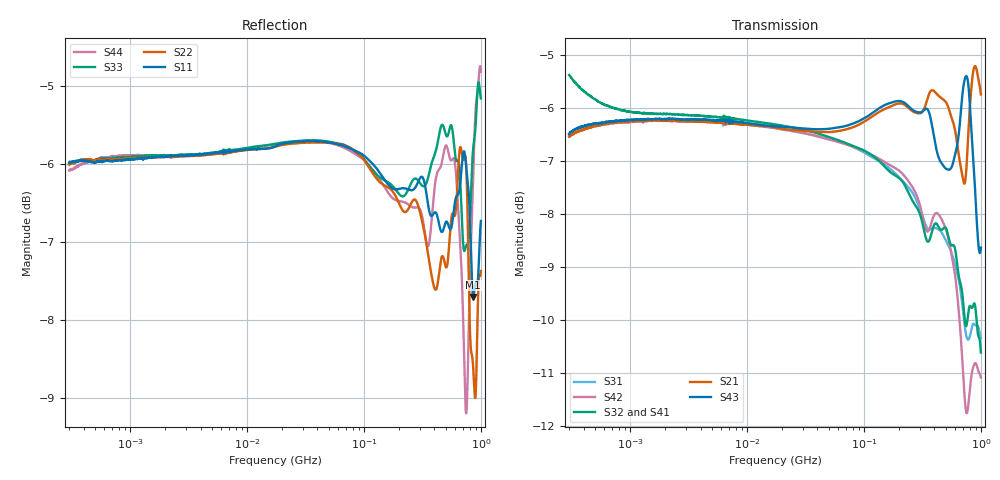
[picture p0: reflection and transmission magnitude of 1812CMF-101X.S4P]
!s-Parameter Generated by FASTRON Sdn. Bhd.
!FASTRON P/N : 1812CMF-101X
!Keysight Technologies: E5071C_MY46733604_B.14.02
!Date: Mon Mar 09 12:42:55 2026
!Version  :Rev00  Mon Mar 09 12:42:55 2026
!Data & Calibration Information:
!Freq	S11:SOLT4(ON)	S12:SOLT4(ON)	S13:SOLT4(ON)	S14:SOLT4(ON)
!	S21:SOLT4(ON)	S22:SOLT4(ON)	S23:SOLT4(ON)	S24:SOLT4(ON)
!	S31:SOLT4(ON)	S32:SOLT4(ON)	S33:SOLT4(ON)	S34:SOLT4(ON)
!	S41:SOLT4(ON)	S42:SOLT4(ON)	S43:SOLT4(ON)	S44:SOLT4(ON)
!PortZ  Port1:50+j0  Port2:50+j0  Port3:50+j0  Port4:50+j0
!When reading reference impedance value at option line is always used.
! Remarks : This data is being provided solely for informational purposes.
# Hz S dB R 50
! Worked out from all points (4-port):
!   1601 points, 300 kHz to 1 GHz, reference 50 ohm
!   strongest paths, dB at 300 kHz, 2.303 MHz, 17.55 MHz, 132.8 MHz, 1 GHz:
!     S43: -6.5, -6.2, -6.3, -6.0, -8.6
!     S21: -6.5, -6.2, -6.4, -6.1, -5.7
!     S32: -5.4, -6.1, -6.3, -7.0, -10.6
!     S41: -5.3, -6.1, -6.3, -7.0, -11.2
!     S42: -6.5, -6.2, -6.4, -6.9, -11.1
!     S31: -6.5, -6.2, -6.4, -7.0, -10.3
!   lowest |S11| = -7.7 dB at 861.1 MHz (marker M1), VSWR 2.40, Z = 120 - j3.58 ohm
!   |S11| at or under -10 dB: nowhere
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300000  -5.98 12.5  -6.57 14.6  -6.54 -165.6  -5.43 -13.5
        -6.54 14.3  -6.01 12.9  -5.37 -13.5  -6.60 -165.5
        -6.52 -165.8  -5.38 -13.5  -6.00 12.8  -6.59 14.6
        -5.33 -13.8  -6.51 -165.8  -6.49 14.3  -6.08 13.7
6.067004e7  -5.75 -4.4  -6.42 0.3  -6.61 152.8  -6.60 -27.2
            -6.43 0.3  -5.74 -6.1  -6.59 -28.0  -6.65 151.7
            -6.63 152.7  -6.61 -28.0  -5.73 -4.9  -6.40 0.4
            -6.59 -27.3  -6.64 151.6  -6.36 0.4  -5.76 -5.3
2.150325e8  -6.31 -10.5  -5.91 -3.1  -7.36 89.4  -7.47 -90.9
            -5.92 -3.0  -6.60 -15.0  -7.38 -92.7  -7.26 86.4
            -7.38 89.5  -7.40 -92.6  -6.41 -10.7  -5.90 -3.5
            -7.47 -90.7  -7.25 86.4  -5.88 -3.7  -6.48 -12.0
4.296107e8  -6.70 -12.5  -5.74 -8.7  -8.26 7.1  -8.25 -174.7
            -5.76 -8.6  -7.51 -17.7  -8.22 -176.4  -8.00 5.7
            -8.28 7.1  -8.22 -176.4  -5.70 -12.2  -6.89 -9.4
            -8.25 -174.6  -7.99 5.8  -6.90 -9.5  -6.09 -11.9
6.319272e8  -6.40 -4.3  -6.72 -15.1  -9.11 -74.8  -8.78 101.8
            -6.73 -15.0  -6.23 -13.6  -9.00 102.7  -9.58 -77.0
            -9.14 -74.8  -9.01 102.6  -5.96 -16.4  -6.62 -2.1
            -8.78 101.9  -9.58 -76.9  -6.66 -2.2  -6.44 -20.8
8.611227e8  -7.71 -1.7  -5.28 -10.5  -10.05 -158.5  -10.40 23.6
            -5.30 -10.4  -8.63 -9.4  -9.72 26.1  -10.90 -155.2
            -10.07 -158.5  -9.72 25.9  -5.78 2.5  -6.97 -19.0
            -10.43 23.8  -10.88 -155.1  -6.96 -19.0  -6.14 4.1
1e9  -6.73 11.3  -5.73 -21.7  -10.34 146.7  -11.19 -29.7
     -5.74 -21.5  -7.37 5.1  -10.63 -30.1  -11.12 145.1
     -10.34 146.7  -10.61 -30.2  -5.16 -7.1  -8.66 -4.4
     -11.21 -29.9  -11.08 145.1  -8.63 -4.2  -4.81 -7.7
